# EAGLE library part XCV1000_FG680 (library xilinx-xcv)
xcv1000_fg680_1532 edit this description Auto generated by make-symbol-device-package-bsdl.ulp Rev. 26 Source: xcv1000_fg680_1532.bsd
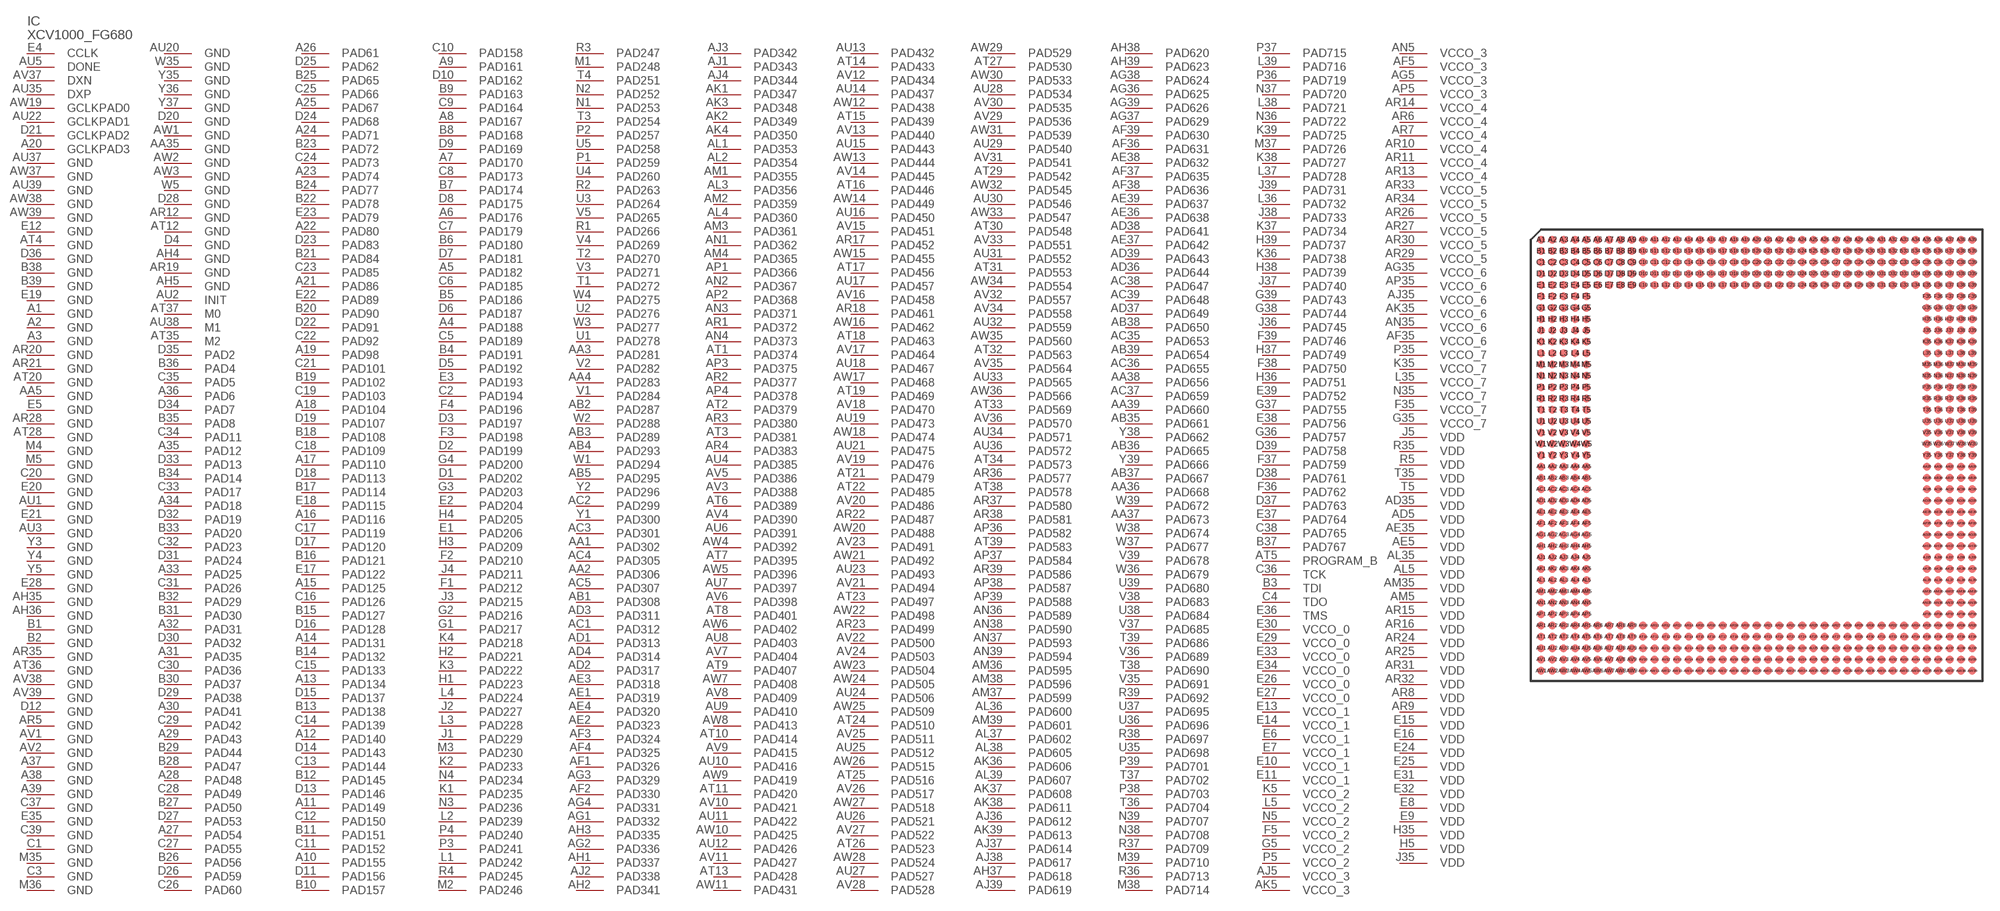
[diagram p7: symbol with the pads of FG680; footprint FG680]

Designator prefix IC

## XCV1000_FG680 (OC_FARNELL: unknown; OC_NEWARK: unknown)  [FG680]
A1  GND  pwr
A2  GND  pwr
A3  GND  pwr
A4  PAD188
A5  PAD182
A6  PAD176
A7  PAD170
A8  PAD167
A9  PAD161
A10  PAD155
A11  PAD149
A12  PAD140
A13  PAD134
A14  PAD131
A15  PAD125
A16  PAD116
A17  PAD110
A18  PAD104
A19  PAD98
A20  GCLKPAD3  in
A21  PAD86
A22  PAD80
A23  PAD74
A24  PAD71
A25  PAD67
A26  PAD61
A27  PAD54
A28  PAD48
A29  PAD43
A30  PAD41
A31  PAD35
A32  PAD31
A33  PAD25
A34  PAD18
A35  PAD12
A36  PAD6
A37  GND  pwr
A38  GND  pwr
A39  GND  pwr
AA1  PAD302
AA2  PAD306
AA3  PAD281
AA4  PAD283
AA5  GND  pwr
AA35  GND  pwr
AA36  PAD668
AA37  PAD673
AA38  PAD656
AA39  PAD660
AB1  PAD308
AB2  PAD287
AB3  PAD289
AB4  PAD293
AB5  PAD295
AB35  PAD661
AB36  PAD665
AB37  PAD667
AB38  PAD650
AB39  PAD654
AC1  PAD312
AC2  PAD299
AC3  PAD301
AC4  PAD305
AC5  PAD307
AC35  PAD653
AC36  PAD655
AC37  PAD659
AC38  PAD647
AC39  PAD648
AD1  PAD313
AD2  PAD317
AD3  PAD311
AD4  PAD314
AD5  VDD  pwr
AD35  VDD  pwr
AD36  PAD644
AD37  PAD649
AD38  PAD641
AD39  PAD643
AE1  PAD319
AE2  PAD323
AE3  PAD318
AE4  PAD320
AE5  VDD  pwr
AE35  VDD  pwr
AE36  PAD638
AE37  PAD642
AE38  PAD632
AE39  PAD637
AF1  PAD326
AF2  PAD330
AF3  PAD324
AF4  PAD325
AF5  VCCO_3  pwr
AF35  VCCO_6  pwr
AF36  PAD631
AF37  PAD635
AF38  PAD636
AF39  PAD630
AG1  PAD332
AG2  PAD336
AG3  PAD329
AG4  PAD331
AG5  VCCO_3  pwr
AG35  VCCO_6  pwr
AG36  PAD625
AG37  PAD629
AG38  PAD624
AG39  PAD626
AH1  PAD337
AH2  PAD341
AH3  PAD335
AH4  GND  pwr
AH5  GND  pwr
AH35  GND  pwr
AH36  GND  pwr
AH37  PAD618
AH38  PAD620
AH39  PAD623
AJ1  PAD343
AJ2  PAD338
AJ3  PAD342
AJ4  PAD344
AJ5  VCCO_3  pwr
AJ35  VCCO_6  pwr
AJ36  PAD612
AJ37  PAD614
AJ38  PAD617
AJ39  PAD619
AK1  PAD347
AK2  PAD349
AK3  PAD348
AK4  PAD350
AK5  VCCO_3  pwr
AK35  VCCO_6  pwr
AK36  PAD606
AK37  PAD608
AK38  PAD611
AK39  PAD613
AL1  PAD353
AL2  PAD354
AL3  PAD356
AL4  PAD360
AL5  VDD  pwr
AL35  VDD  pwr
AL36  PAD600
AL37  PAD602
AL38  PAD605
AL39  PAD607
AM1  PAD355
AM2  PAD359
AM3  PAD361
AM4  PAD365
AM5  VDD  pwr
AM35  VDD  pwr
AM36  PAD595
AM37  PAD599
AM38  PAD596
AM39  PAD601
AN1  PAD362
AN2  PAD367
AN3  PAD371
AN4  PAD373
AN5  VCCO_3  pwr
AN35  VCCO_6  pwr
AN36  PAD589
AN37  PAD593
AN38  PAD590
AN39  PAD594
AP1  PAD366
AP2  PAD368
AP3  PAD375
AP4  PAD378
AP5  VCCO_3  pwr
AP35  VCCO_6  pwr
AP36  PAD582
AP37  PAD584
AP38  PAD587
AP39  PAD588
AR1  PAD372
AR2  PAD377
AR3  PAD380
AR4  PAD383
AR5  GND  pwr
AR6  VCCO_4  pwr
AR7  VCCO_4  pwr
AR8  VDD  pwr
AR9  VDD  pwr
AR10  VCCO_4  pwr
AR11  VCCO_4  pwr
AR12  GND  pwr
AR13  VCCO_4  pwr
AR14  VCCO_4  pwr
AR15  VDD  pwr
AR16  VDD  pwr
AR17  PAD452
AR18  PAD461
AR19  GND  pwr
AR20  GND  pwr
AR21  GND  pwr
AR22  PAD487
AR23  PAD499
AR24  VDD  pwr
AR25  VDD  pwr
AR26  VCCO_5  pwr
AR27  VCCO_5  pwr
AR28  GND  pwr
AR29  VCCO_5  pwr
AR30  VCCO_5  pwr
AR31  VDD  pwr
AR32  VDD  pwr
AR33  VCCO_5  pwr
AR34  VCCO_5  pwr
AR35  GND  pwr
AR36  PAD577
AR37  PAD580
AR38  PAD581
AR39  PAD586
AT1  PAD374
AT2  PAD379
AT3  PAD381
AT4  GND  pwr
AT5  PROGRAM_B  in
AT6  PAD389
AT7  PAD395
AT8  PAD401
AT9  PAD407
AT10  PAD414
AT11  PAD420
AT12  GND  pwr
AT13  PAD428
AT14  PAD433
AT15  PAD439
AT16  PAD446
AT17  PAD456
AT18  PAD463
AT19  PAD469
AT20  GND  pwr
AT21  PAD479
AT22  PAD485
AT23  PAD497
AT24  PAD510
AT25  PAD516
AT26  PAD523
AT27  PAD530
AT28  GND  pwr
AT29  PAD542
AT30  PAD548
AT31  PAD553
AT32  PAD563
AT33  PAD569
AT34  PAD573
AT35  M2  in
AT36  GND  pwr
AT37  M0  in
AT38  PAD578
AT39  PAD583
AU1  GND  pwr
AU2  INIT
AU3  GND  pwr
AU4  PAD385
AU5  DONE
AU6  PAD391
AU7  PAD397
AU8  PAD403
AU9  PAD410
AU10  PAD416
AU11  PAD422
AU12  PAD426
AU13  PAD432
AU14  PAD437
AU15  PAD443
AU16  PAD450
AU17  PAD457
AU18  PAD467
AU19  PAD473
AU20  GND  pwr
AU21  PAD475
AU22  GCLKPAD1  in
AU23  PAD493
AU24  PAD506
AU25  PAD512
AU26  PAD521
AU27  PAD527
AU28  PAD534
AU29  PAD540
AU30  PAD546
AU31  PAD552
AU32  PAD559
AU33  PAD565
AU34  PAD571
AU35  DXP  pas
AU36  PAD572
AU37  GND  pwr
AU38  M1  in
AU39  GND  pwr
AV1  GND  pwr
AV2  GND  pwr
AV3  PAD388
AV4  PAD390
AV5  PAD386
AV6  PAD398
AV7  PAD404
AV8  PAD409
AV9  PAD415
AV10  PAD421
AV11  PAD427
AV12  PAD434
AV13  PAD440
AV14  PAD445
AV15  PAD451
AV16  PAD458
AV17  PAD464
AV18  PAD470
AV19  PAD476
AV20  PAD486
AV21  PAD494
AV22  PAD500
AV23  PAD491
AV24  PAD503
AV25  PAD511
AV26  PAD517
AV27  PAD522
AV28  PAD528
AV29  PAD536
AV30  PAD535
AV31  PAD541
AV32  PAD557
AV33  PAD551
AV34  PAD558
AV35  PAD564
AV36  PAD570
AV37  DXN  pas
AV38  GND  pwr
AV39  GND  pwr
AW1  GND  pwr
AW2  GND  pwr
AW3  GND  pwr
AW4  PAD392
AW5  PAD396
AW6  PAD402
AW7  PAD408
AW8  PAD413
AW9  PAD419
AW10  PAD425
AW11  PAD431
AW12  PAD438
AW13  PAD444
AW14  PAD449
AW15  PAD455
AW16  PAD462
AW17  PAD468
AW18  PAD474
AW19  GCLKPAD0  in
AW20  PAD488
AW21  PAD492
AW22  PAD498
AW23  PAD504
AW24  PAD505
AW25  PAD509
AW26  PAD515
AW27  PAD518
AW28  PAD524
AW29  PAD529
AW30  PAD533
AW31  PAD539
AW32  PAD545
AW33  PAD547
AW34  PAD554
AW35  PAD560
AW36  PAD566
AW37  GND  pwr
AW38  GND  pwr
AW39  GND  pwr
B1  GND  pwr
B2  GND  pwr
B3  TDI  in
B4  PAD191
B5  PAD186
B6  PAD180
B7  PAD174
B8  PAD168
B9  PAD163
B10  PAD157
B11  PAD151
B12  PAD145
B13  PAD138
B14  PAD132
B15  PAD127
B16  PAD121
B17  PAD114
B18  PAD108
B19  PAD102
B20  PAD90
B21  PAD84
B22  PAD78
B23  PAD72
B24  PAD77
B25  PAD65
B26  PAD56
B27  PAD50
B28  PAD47
B29  PAD44
B30  PAD37
B31  PAD30
B32  PAD29
B33  PAD20
B34  PAD14
B35  PAD8
B36  PAD4
B37  PAD767
B38  GND  pwr
B39  GND  pwr
C1  GND  pwr
C2  PAD194
C3  GND  pwr
C4  TDO  out
C5  PAD189
C6  PAD185
C7  PAD179
C8  PAD173
C9  PAD164
C10  PAD158
C11  PAD152
C12  PAD150
C13  PAD144
C14  PAD139
C15  PAD133
C16  PAD126
C17  PAD119
C18  PAD109
C19  PAD103
C20  GND  pwr
C21  PAD101
C22  PAD92
C23  PAD85
C24  PAD73
C25  PAD66
C26  PAD60
C27  PAD55
C28  PAD49
C29  PAD42
C30  PAD36
C31  PAD26
C32  PAD23
C33  PAD17
C34  PAD11
C35  PAD5
C36  TCK  in
C37  GND  pwr
C38  PAD765
C39  GND  pwr
D1  PAD202
D2  PAD199
D3  PAD197
D4  GND  pwr
D5  PAD192
D6  PAD187
D7  PAD181
D8  PAD175
D9  PAD169
D10  PAD162
D11  PAD156
D12  GND  pwr
D13  PAD146
D14  PAD143
D15  PAD137
D16  PAD128
D17  PAD120
D18  PAD113
D19  PAD107
D20  GND  pwr
D21  GCLKPAD2  in
D22  PAD91
D23  PAD83
D24  PAD68
D25  PAD62
D26  PAD59
D27  PAD53
D28  GND  pwr
D29  PAD38
D30  PAD32
D31  PAD24
D32  PAD19
D33  PAD13
D34  PAD7
D35  PAD2
D36  GND  pwr
D37  PAD763
D38  PAD761
D39  PAD758
E1  PAD206
E2  PAD204
E3  PAD193
E4  CCLK
E5  GND  pwr
E6  VCCO_1  pwr
E7  VCCO_1  pwr
E8  VDD  pwr
E9  VDD  pwr
E10  VCCO_1  pwr
E11  VCCO_1  pwr
E12  GND  pwr
E13  VCCO_1  pwr
E14  VCCO_1  pwr
E15  VDD  pwr
E16  VDD  pwr
E17  PAD122
E18  PAD115
E19  GND  pwr
E20  GND  pwr
E21  GND  pwr
E22  PAD89
E23  PAD79
E24  VDD  pwr
E25  VDD  pwr
E26  VCCO_0  pwr
E27  VCCO_0  pwr
E28  GND  pwr
E29  VCCO_0  pwr
E30  VCCO_0  pwr
E31  VDD  pwr
E32  VDD  pwr
E33  VCCO_0  pwr
E34  VCCO_0  pwr
E35  GND  pwr
E36  TMS  in
E37  PAD764
E38  PAD756
E39  PAD752
F1  PAD212
F2  PAD210
F3  PAD198
F4  PAD196
F5  VCCO_2  pwr
F35  VCCO_7  pwr
F36  PAD762
F37  PAD759
F38  PAD750
F39  PAD746
G1  PAD217
G2  PAD216
G3  PAD203
G4  PAD200
G5  VCCO_2  pwr
G35  VCCO_7  pwr
G36  PAD757
G37  PAD755
G38  PAD744
G39  PAD743
H1  PAD223
H2  PAD221
H3  PAD209
H4  PAD205
H5  VDD  pwr
H35  VDD  pwr
H36  PAD751
H37  PAD749
H38  PAD739
H39  PAD737
J1  PAD229
J2  PAD227
J3  PAD215
J4  PAD211
J5  VDD  pwr
J35  VDD  pwr
J36  PAD745
J37  PAD740
J38  PAD733
J39  PAD731
K1  PAD235
K2  PAD233
K3  PAD222
K4  PAD218
K5  VCCO_2  pwr
K35  VCCO_7  pwr
K36  PAD738
K37  PAD734
K38  PAD727
K39  PAD725
L1  PAD242
L2  PAD239
L3  PAD228
L4  PAD224
L5  VCCO_2  pwr
L35  VCCO_7  pwr
L36  PAD732
L37  PAD728
L38  PAD721
L39  PAD716
M1  PAD248
M2  PAD246
M3  PAD230
M4  GND  pwr
M5  GND  pwr
M35  GND  pwr
M36  GND  pwr
M37  PAD726
M38  PAD714
M39  PAD710
N1  PAD253
N2  PAD252
N3  PAD236
N4  PAD234
N5  VCCO_2  pwr
N35  VCCO_7  pwr
N36  PAD722
N37  PAD720
N38  PAD708
N39  PAD707
P1  PAD259
P2  PAD257
P3  PAD241
P4  PAD240
P5  VCCO_2  pwr
P35  VCCO_7  pwr
P36  PAD719
P37  PAD715
P38  PAD703
P39  PAD701
R1  PAD266
R2  PAD263
R3  PAD247
R4  PAD245
R5  VDD  pwr
R35  VDD  pwr
R36  PAD713
R37  PAD709
R38  PAD697
R39  PAD692
T1  PAD272
T2  PAD270
T3  PAD254
T4  PAD251
T5  VDD  pwr
T35  VDD  pwr
T36  PAD704
T37  PAD702
T38  PAD690
T39  PAD686
U1  PAD278
U2  PAD276
U3  PAD264
U4  PAD260
U5  PAD258
U35  PAD698
U36  PAD696
U37  PAD695
U38  PAD684
U39  PAD680
V1  PAD284
V2  PAD282
V3  PAD271
V4  PAD269
V5  PAD265
V35  PAD691
V36  PAD689
V37  PAD685
V38  PAD683
V39  PAD678
W1  PAD294
W2  PAD288
W3  PAD277
W4  PAD275
W5  GND  pwr
W35  GND  pwr
W36  PAD679
W37  PAD677
W38  PAD674
W39  PAD672
Y1  PAD300
Y2  PAD296
Y3  GND  pwr
Y4  GND  pwr
Y5  GND  pwr
Y35  GND  pwr
Y36  GND  pwr
Y37  GND  pwr
Y38  PAD662
Y39  PAD666

## Footprint FG680 (pad centres in mm)
xcv1000_fg680_1532 edit this description Auto generated by make-symbol-device-package-bsdl.ulp Rev. 26 Source: xcv1000_fg680_1532.bsd
smd 0.7 x 0.7: A1 -19,19; A2 -18,19; A3 -17,19; A4 -16,19; A5 -15,19; A6 -14,19; A7 -13,19; A8 -12,19; A9 -11,19; A10 -10,19; A11 -9,19; A12 -8,19; A13 -7,19; A14 -6,19; A15 -5,19; A16 -4,19; A17 -3,19; A18 -2,19; A19 -1,19; A20 0,19; A21 1,19; A22 2,19; A23 3,19; A24 4,19; A25 5,19; A26 6,19; A27 7,19; A28 8,19; A29 9,19; A30 10,19; A31 11,19; A32 12,19; A33 13,19; A34 14,19; A35 15,19; A36 16,19; A37 17,19; A38 18,19; A39 19,19; AA1 -19,-1; AA2 -18,-1; AA3 -17,-1; AA4 -16,-1; AA5 -15,-1; AA35 15,-1; AA36 16,-1; AA37 17,-1; AA38 18,-1; AA39 19,-1; AB1 -19,-2; AB2 -18,-2; AB3 -17,-2; AB4 -16,-2; AB5 -15,-2; AB35 15,-2; AB36 16,-2; AB37 17,-2; AB38 18,-2; AB39 19,-2; AC1 -19,-3; AC2 -18,-3; AC3 -17,-3; AC4 -16,-3; AC5 -15,-3; AC35 15,-3; AC36 16,-3; AC37 17,-3; AC38 18,-3; AC39 19,-3; AD1 -19,-4; AD2 -18,-4; AD3 -17,-4; AD4 -16,-4; AD5 -15,-4; AD35 15,-4; AD36 16,-4; AD37 17,-4; AD38 18,-4; AD39 19,-4; AE1 -19,-5; AE2 -18,-5; AE3 -17,-5; AE4 -16,-5; AE5 -15,-5; AE35 15,-5; AE36 16,-5; AE37 17,-5; AE38 18,-5; AE39 19,-5; AF1 -19,-6; AF2 -18,-6; AF3 -17,-6; AF4 -16,-6; AF5 -15,-6; AF35 15,-6; AF36 16,-6; AF37 17,-6; AF38 18,-6; AF39 19,-6; AG1 -19,-7; AG2 -18,-7; AG3 -17,-7; AG4 -16,-7; AG5 -15,-7; AG35 15,-7; AG36 16,-7; AG37 17,-7; AG38 18,-7; AG39 19,-7; AH1 -19,-8; AH2 -18,-8; AH3 -17,-8; AH4 -16,-8; AH5 -15,-8; AH35 15,-8; AH36 16,-8; AH37 17,-8; AH38 18,-8; AH39 19,-8; AJ1 -19,-9; AJ2 -18,-9; AJ3 -17,-9; AJ4 -16,-9; AJ5 -15,-9; AJ35 15,-9; AJ36 16,-9; AJ37 17,-9; AJ38 18,-9; AJ39 19,-9; AK1 -19,-10; AK2 -18,-10; AK3 -17,-10; AK4 -16,-10; AK5 -15,-10; AK35 15,-10; AK36 16,-10; AK37 17,-10; AK38 18,-10; AK39 19,-10; AL1 -19,-11; AL2 -18,-11; AL3 -17,-11; AL4 -16,-11; AL5 -15,-11; AL35 15,-11; AL36 16,-11; AL37 17,-11; AL38 18,-11; AL39 19,-11; AM1 -19,-12; AM2 -18,-12; AM3 -17,-12; AM4 -16,-12; AM5 -15,-12; AM35 15,-12; AM36 16,-12; AM37 17,-12; AM38 18,-12; AM39 19,-12; AN1 -19,-13; AN2 -18,-13; AN3 -17,-13; AN4 -16,-13; AN5 -15,-13; AN35 15,-13; AN36 16,-13; AN37 17,-13; AN38 18,-13; AN39 19,-13; AP1 -19,-14; AP2 -18,-14; AP3 -17,-14; AP4 -16,-14; AP5 -15,-14; AP35 15,-14; AP36 16,-14; AP37 17,-14; AP38 18,-14; AP39 19,-14; AR1 -19,-15; AR2 -18,-15; AR3 -17,-15; AR4 -16,-15; AR5 -15,-15; AR6 -14,-15; AR7 -13,-15; AR8 -12,-15; AR9 -11,-15; AR10 -10,-15; AR11 -9,-15; AR12 -8,-15; AR13 -7,-15; AR14 -6,-15; AR15 -5,-15; AR16 -4,-15; AR17 -3,-15; AR18 -2,-15; AR19 -1,-15; AR20 0,-15; AR21 1,-15; AR22 2,-15; AR23 3,-15; AR24 4,-15; AR25 5,-15; AR26 6,-15; AR27 7,-15; AR28 8,-15; AR29 9,-15; AR30 10,-15; AR31 11,-15; AR32 12,-15; AR33 13,-15; AR34 14,-15; AR35 15,-15; AR36 16,-15; AR37 17,-15; AR38 18,-15; AR39 19,-15; AT1 -19,-16; AT2 -18,-16; AT3 -17,-16; AT4 -16,-16; AT5 -15,-16; AT6 -14,-16; AT7 -13,-16; AT8 -12,-16; AT9 -11,-16; AT10 -10,-16; AT11 -9,-16; AT12 -8,-16; AT13 -7,-16; AT14 -6,-16; AT15 -5,-16; AT16 -4,-16; AT17 -3,-16; AT18 -2,-16; AT19 -1,-16; AT20 0,-16; AT21 1,-16; AT22 2,-16; AT23 3,-16; AT24 4,-16; AT25 5,-16; AT26 6,-16; AT27 7,-16; AT28 8,-16; AT29 9,-16; AT30 10,-16; AT31 11,-16; AT32 12,-16; AT33 13,-16; AT34 14,-16; AT35 15,-16; AT36 16,-16; AT37 17,-16; AT38 18,-16; AT39 19,-16; AU1 -19,-17; AU2 -18,-17; AU3 -17,-17; AU4 -16,-17; AU5 -15,-17; AU6 -14,-17; AU7 -13,-17; AU8 -12,-17; AU9 -11,-17; AU10 -10,-17; AU11 -9,-17; AU12 -8,-17; AU13 -7,-17; AU14 -6,-17; AU15 -5,-17; AU16 -4,-17; AU17 -3,-17; AU18 -2,-17; AU19 -1,-17; AU20 0,-17; AU21 1,-17; AU22 2,-17; AU23 3,-17; AU24 4,-17; AU25 5,-17; AU26 6,-17; AU27 7,-17; AU28 8,-17; AU29 9,-17; AU30 10,-17; AU31 11,-17; AU32 12,-17; AU33 13,-17; AU34 14,-17; AU35 15,-17; AU36 16,-17; AU37 17,-17; AU38 18,-17; AU39 19,-17; AV1 -19,-18; AV2 -18,-18; AV3 -17,-18; AV4 -16,-18; AV5 -15,-18; AV6 -14,-18; AV7 -13,-18; AV8 -12,-18; AV9 -11,-18; AV10 -10,-18; AV11 -9,-18; AV12 -8,-18; AV13 -7,-18; AV14 -6,-18; AV15 -5,-18; AV16 -4,-18; AV17 -3,-18; AV18 -2,-18; AV19 -1,-18; AV20 0,-18; AV21 1,-18; AV22 2,-18; AV23 3,-18; AV24 4,-18; AV25 5,-18; AV26 6,-18; AV27 7,-18; AV28 8,-18; AV29 9,-18; AV30 10,-18; AV31 11,-18; AV32 12,-18; AV33 13,-18; AV34 14,-18; AV35 15,-18; AV36 16,-18; AV37 17,-18; AV38 18,-18; AV39 19,-18; AW1 -19,-19; AW2 -18,-19; AW3 -17,-19; AW4 -16,-19; AW5 -15,-19; AW6 -14,-19; AW7 -13,-19; AW8 -12,-19; AW9 -11,-19; AW10 -10,-19; AW11 -9,-19; AW12 -8,-19; AW13 -7,-19; AW14 -6,-19; AW15 -5,-19; AW16 -4,-19; AW17 -3,-19; AW18 -2,-19; AW19 -1,-19; AW20 0,-19; AW21 1,-19; AW22 2,-19; AW23 3,-19; AW24 4,-19; AW25 5,-19; AW26 6,-19; AW27 7,-19; AW28 8,-19; AW29 9,-19; AW30 10,-19; AW31 11,-19; AW32 12,-19; AW33 13,-19; AW34 14,-19; AW35 15,-19; AW36 16,-19; AW37 17,-19; AW38 18,-19; AW39 19,-19; B1 -19,18; B2 -18,18; B3 -17,18; B4 -16,18; B5 -15,18; B6 -14,18; B7 -13,18; B8 -12,18; B9 -11,18; B10 -10,18; B11 -9,18; B12 -8,18; B13 -7,18; B14 -6,18; B15 -5,18; B16 -4,18; B17 -3,18; B18 -2,18; B19 -1,18; B20 0,18; B21 1,18; B22 2,18; B23 3,18; B24 4,18; B25 5,18; B26 6,18; B27 7,18; B28 8,18; B29 9,18; B30 10,18; B31 11,18; B32 12,18; B33 13,18; B34 14,18; B35 15,18; B36 16,18; B37 17,18; B38 18,18; B39 19,18; C1 -19,17; C2 -18,17; C3 -17,17; C4 -16,17; C5 -15,17; C6 -14,17; C7 -13,17; C8 -12,17; C9 -11,17; C10 -10,17; C11 -9,17; C12 -8,17; C13 -7,17; C14 -6,17; C15 -5,17; C16 -4,17; C17 -3,17; C18 -2,17; C19 -1,17; C20 0,17; C21 1,17; C22 2,17; C23 3,17; C24 4,17; C25 5,17; C26 6,17; C27 7,17; C28 8,17; C29 9,17; C30 10,17; C31 11,17; C32 12,17; C33 13,17; C34 14,17; C35 15,17; C36 16,17; C37 17,17; C38 18,17; C39 19,17; D1 -19,16; D2 -18,16; D3 -17,16; D4 -16,16; D5 -15,16; D6 -14,16; D7 -13,16; D8 -12,16; D9 -11,16; D10 -10,16; D11 -9,16; D12 -8,16; D13 -7,16; D14 -6,16; D15 -5,16; D16 -4,16; D17 -3,16; D18 -2,16; D19 -1,16; D20 0,16; D21 1,16; D22 2,16; D23 3,16; D24 4,16; D25 5,16; D26 6,16; D27 7,16; D28 8,16; D29 9,16; D30 10,16; D31 11,16; D32 12,16; D33 13,16; D34 14,16; D35 15,16; D36 16,16; D37 17,16; D38 18,16; D39 19,16; E1 -19,15; E2 -18,15; E3 -17,15; E4 -16,15; E5 -15,15; E6 -14,15; E7 -13,15; E8 -12,15; E9 -11,15; E10 -10,15; E11 -9,15; E12 -8,15; E13 -7,15; E14 -6,15; E15 -5,15; E16 -4,15; E17 -3,15; E18 -2,15; E19 -1,15; E20 0,15; E21 1,15; E22 2,15; E23 3,15; E24 4,15; E25 5,15; E26 6,15; E27 7,15; E28 8,15; E29 9,15; E30 10,15; E31 11,15; E32 12,15; E33 13,15; E34 14,15; E35 15,15; E36 16,15; E37 17,15; E38 18,15; E39 19,15; F1 -19,14; F2 -18,14; F3 -17,14; F4 -16,14; F5 -15,14; F35 15,14; F36 16,14; F37 17,14; F38 18,14; F39 19,14; G1 -19,13; G2 -18,13; G3 -17,13; G4 -16,13; G5 -15,13; G35 15,13; G36 16,13; G37 17,13; G38 18,13; G39 19,13; H1 -19,12; H2 -18,12; H3 -17,12; H4 -16,12; H5 -15,12; H35 15,12; H36 16,12; H37 17,12; H38 18,12; H39 19,12; J1 -19,11; J2 -18,11; J3 -17,11; J4 -16,11; J5 -15,11; J35 15,11; J36 16,11; J37 17,11; J38 18,11; J39 19,11; K1 -19,10; K2 -18,10; K3 -17,10; K4 -16,10; K5 -15,10; K35 15,10; K36 16,10; K37 17,10; K38 18,10; K39 19,10; L1 -19,9; L2 -18,9; L3 -17,9; L4 -16,9; L5 -15,9; L35 15,9; L36 16,9; L37 17,9; L38 18,9; L39 19,9; M1 -19,8; M2 -18,8; M3 -17,8; M4 -16,8; M5 -15,8; M35 15,8; M36 16,8; M37 17,8; M38 18,8; M39 19,8; N1 -19,7; N2 -18,7; N3 -17,7; N4 -16,7; N5 -15,7; N35 15,7; N36 16,7; N37 17,7; N38 18,7; N39 19,7; P1 -19,6; P2 -18,6; P3 -17,6; P4 -16,6; P5 -15,6; P35 15,6; P36 16,6; P37 17,6; P38 18,6; P39 19,6; R1 -19,5; R2 -18,5; R3 -17,5; R4 -16,5; R5 -15,5; R35 15,5; R36 16,5; R37 17,5; R38 18,5; R39 19,5; T1 -19,4; T2 -18,4; T3 -17,4; T4 -16,4; T5 -15,4; T35 15,4; T36 16,4; T37 17,4; T38 18,4; T39 19,4; U1 -19,3; U2 -18,3; U3 -17,3; U4 -16,3; U5 -15,3; U35 15,3; U36 16,3; U37 17,3; U38 18,3; U39 19,3; V1 -19,2; V2 -18,2; V3 -17,2; V4 -16,2; V5 -15,2; V35 15,2; V36 16,2; V37 17,2; V38 18,2; V39 19,2; W1 -19,1; W2 -18,1; W3 -17,1; W4 -16,1; W5 -15,1; W35 15,1; W36 16,1; W37 17,1; W38 18,1; W39 19,1; Y1 -19,0; Y2 -18,0; Y3 -17,0; Y4 -16,0; Y5 -15,0; Y35 15,0; Y36 16,0; Y37 17,0; Y38 18,0; Y39 19,0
